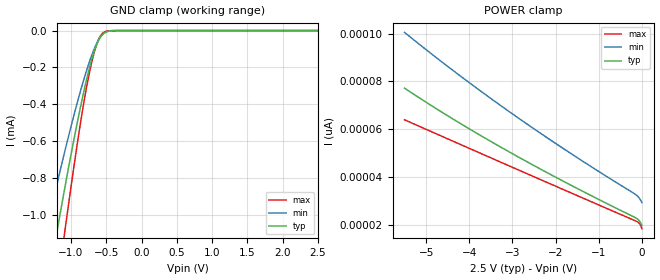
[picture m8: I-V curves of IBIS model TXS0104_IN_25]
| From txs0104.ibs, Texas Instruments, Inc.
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[Model]   TXS0104_IN_25
Model_type  Input
Vinl=0.7
Vinh=1.7
| variable   typ   min   max
C_comp   0.22pF   0.17pF   0.26pF
[Temperature Range]   40   100   -40
| Ambient temperature   25   85   -40
[Voltage range]   2.5   2.3   2.7
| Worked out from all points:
|   GND clamp passes 1 mA (typ) near -1.16 V on its own axis
[GND Clamp]
| TXS0104_IN_25
|   Voltage   I(typ)   I(min)   I(max)
-5.5V     -12.44mA   -9.732mA   -15.69mA
-1.395V   -1.529mA   -1.163mA   -1.988mA
-1.345V   -1.415mA   -1.077mA   -1.838mA
-1.2V     -1.093mA   -834.5uA   -1.41mA
-1.11V    -899.7uA   -689.7uA   -1.152mA
-1.07V    -816uA     -627uA     -1.04mA
-880mV    -440.9uA   -347.4uA   -536.3uA
-755mV    -226.3uA   -187.7uA   -258.9uA
-640mV    -79.19uA   -72.62uA   -78.88uA
-550mV    -20.17uA   -19.87uA   -13.42uA
-385mV    -371.3nA   -510.2nA   -61.3nA
2.5V      19.67pA    33.3pA     15.01pA
[POWER Clamp]
| TXS0104_IN_25
|   Voltage   I(typ)   I(min)   I(max)
-5.5V     77.19pA    100.5pA    63.95pA
-4.265V   63.03pA    83.07pA    54.09pA
-2.965V   49.39pA    65.98pA    43.77pA
-1.64V    36.51pA    49.76pA    33.31pA
-140mV    22.83pA    32.57pA    21.54pA
-55mV     21.53pA    31pA       20.51pA
-30mV     20.79pA    30.28pA    19.76pA
-95.1fV   19.67pA    29.27pA    18.35pA
